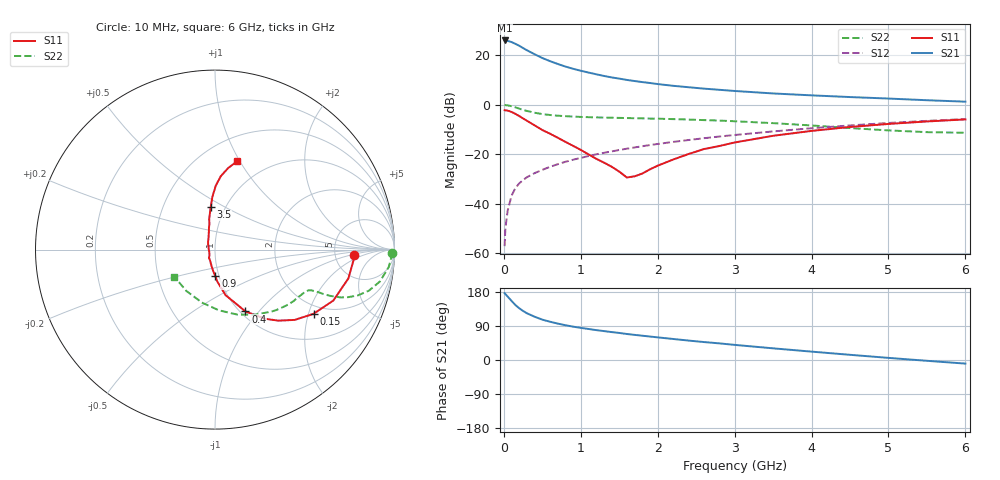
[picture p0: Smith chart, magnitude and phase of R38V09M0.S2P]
! SIEMENS Small Signal Semiconductors
! BFR181
! Si NPN RF Bipolar Junction Transistor in SOT23
! VCE = 8 V  IC = 9 mA
! Common Emitter S-Parameters:  May  1996
# GHz  S  MA  R  50
!  f  S11  S21  S12  S22
! GHz  MAG  ANG  MAG  ANG  MAG  ANG  MAG  ANG
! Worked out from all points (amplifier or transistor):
!   36 points, 10 MHz to 6 GHz, reference 50 ohm
!   highest |S21| = 26.0 dB at 10 MHz (marker M1)
!   |S21| within 3 dB of that: start of sweep to 246.3 MHz
!   unconditionally stable (mu >= 1): 922.8 MHz to 2.85 GHz
!   at 250 MHz: K = 0.56, MSG = 26.6 dB, |S12| = -30.4 dB
!   at 1.4 GHz: K = 1.05, MAG = 13.6 dB, |S12| = -18.8 dB
!   at 6 GHz: K = 0.86, MSG = 3.5 dB, |S12| = -5.8 dB
!   S11 on the Smith chart (normalised r, x): 10 MHz: 7.78, -1.22; 150 MHz: 1.72, -2.16; 400 MHz: 1.05, -0.85; 900 MHz: 0.96, -0.29; 3.5 GHz: 0.85, +0.43; 6 GHz: 0.74, +0.97
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0.01  0.7771 -2.3  19.86 176.4  0.0014 91.6  0.9851 -1.0
0.02  0.7733 -4.6  19.52 174.1  0.0032 85.7  0.9843 -2.3
0.05  0.7602 -12.2  19.46 167.3  0.0073 83.5  0.9726 -5.8
0.1  0.7178 -23.3  18.43 156.0  0.0146 78.0  0.9354 -11.0
0.15  0.6551 -33.1  16.97 145.1  0.0208 73.3  0.8867 -15.0
0.2  0.5923 -41.4  15.52 136.6  0.0259 72.0  0.8353 -17.8
0.25  0.5302 -48.3  13.95 129.4  0.0302 69.3  0.7893 -19.6
0.3  0.4759 -54.1  12.6 123.3  0.0345 69.0  0.7511 -20.8
0.4  0.3839 -63.8  10.47 114.2  0.0417 67.6  0.6909 -21.9
0.5  0.3093 -70.2  8.787 106.5  0.0486 68.2  0.6487 -22.3
0.6  0.2607 -77.0  7.593 101.0  0.0559 68.2  0.6218 -22.4
0.7  0.2167 -80.8  6.667 96.1  0.0631 68.5  0.6023 -22.7
0.9  0.1484 -89.3  5.325 88.0  0.0778 68.3  0.5772 -23.1
1.1  0.0997 -99.9  4.472 81.9  0.0922 68.8  0.5621 -24.2
1.3  0.0681 -113.0  3.821 76.3  0.1071 68.3  0.5513 -25.6
1.6  0.034 -162.5  3.17 68.6  0.13 67.4  0.5392 -28.5
2.2  0.0784 117.2  2.415 55.5  0.1778 64.1  0.5136 -35.8
2.6  0.1275 105.2  2.118 47.4  0.2112 61.4  0.4904 -41.6
3.5  0.2366 95.9  1.692 30.8  0.2897 53.7  0.4257 -58.3
4.5  0.3561 89.3  1.431 13.7  0.383 43.2  0.3385 -86.5
5.5  0.4604 80.8  1.235 -2.1  0.4731 30.9  0.2802 -124.8
6  0.5064 76.0  1.155 -9.5  0.5153 24.2  0.2723 -146.5
